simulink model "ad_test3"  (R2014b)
settings: Solver=ode45  StartTime=0.0  StopTime=10  MaxStep=1e-4  RelTol=1e-3
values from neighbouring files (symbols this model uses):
  ampl = 1    [abtast_rate_1.m]    (also in ad_test_12.m; ad_test_2.m; ad_test_3.m; fft_1.m = 10)
  ampl1 = 1e-4    (= 0.0001)    [ad_test_2.m]    (also in ad_test_3.m; DA_wandler_spektr_1.m = 1; DA_wandler_spektr_2.m = 1; fourier_reihe1.m = 5)
  ampl2 = 1e-5    (= 1e-05)    [ad_test_2.m]    (also in ad_test_3.m; DA_wandler_spektr_1.m = 1; DA_wandler_spektr_2.m = 1; fourier_reihe1.m = 12)
  fsig = 100    [abtast_rate_1.m]    (also in ad_test_12.m = ',num2str(fsig),'; ad_test_2.m = ',num2str(fsig),'; ad_test_3.m = ',num2str(fsig),'; leakage_2.m = 100.5)
  N = 4*1024    (= 4096)    [ad_test_12.m]    (also in ad_test_2.m; ad_test_3.m; DA_wandler_spektr_1.m = 1000; DA_wandler_spektr_2.m = 1024)
  Ts = 1/fs    (= 0.00025)    [abtast_rate_1.m]    (also in ad_test_12.m = 0.0009765625; ad_test_2.m = 0.00048828125; ad_test_3.m = 0.00048828125; DA_wandler_spektr_1.m = 0.01)
undefined symbols (not defined in the file or in its folder): get
libraries: dspspect3 x1, dspstat3 x1, dspsnks4 x1, dspsigops x1

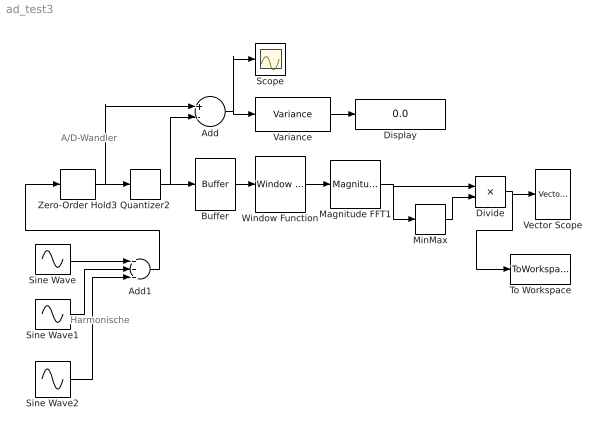
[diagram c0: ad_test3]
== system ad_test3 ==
  note: Harmonische
  note: A/D-Wandler
  Add : Sum  Inputs=+-
  Add1 : Sum  Inputs=+++  SampleTime=0
  Buffer : Buffer  N=N  TreatMby1Signals=One channel
  Display : Display
  Divide : Product  Inputs=*/
  Magnitude FFT1 : dspspect3/Magnitude FFT  mag_or_magsq=Magnitude squared  FFTImplementation=FFTW  fftLenInherit=off  fftsize=N  WrapInput=on
  MinMax : MinMax  Function=max  OutDataTypeStr=double
  Quantizer2 : Quantizer  QuantizationInterval=q  LinearizeAsGain=off  SampleTime=Ts
  Scope : Scope
  Sine Wave : Sin  Amplitude=ampl  Frequency=2*pi*fsig  SampleTime=0
  Sine Wave1 : Sin  Amplitude=ampl1  Frequency=2*pi*[2*fsig]  SampleTime=0
  Sine Wave2 : Sin  Amplitude=ampl2  Frequency=2*pi*[3*fsig]  SampleTime=0
  To Workspace : ToWorkspace  VariableName=Y  SampleTime=-1
  Variance : dspstat3/Variance  run=on  reset_popup=None  InputProcessing=Columns as channels (frame based)  directionMode=Each column  dimension=1  treatSBRowAsCol=on  roiEnable=off  roiType=Rectangles  roiPortion=Entire ROI  roiOutput=Individual statistics for each ROI  roiFlag=off  roundingMode=Floor  overflowMode=off
  Vector Scope : dspsnks4/Vector Scope  ScopeProperties=on  Domain=Frequency  HorizSpan=1  DisplayProperties=off  AxisGrid=on  Memory=off  FrameNumber=on  AxisLegend=off  AxisZoom=off  OpenScopeAtSimStart=on  OpenScopeImmediately=off  FigPos=get(0,'defaultfigureposition')  AxisProperties=off  XUnits=Hertz  XRange=[0...Fs]  InheritXIncr=on  XIncr=1  XLabel=Time  XLimit=User-defined  XMin=2.1333  XMax=2050.1333  XStart=0  YUnits=dB  YLabel=Leistung in dB  LineProperties=off  XAxisParamsVer=6.9
  Window Function : dspsigops/Window Function  winmode=Apply window to input  wintype=Hanning  sampmode=Continuous  samptime=1  N=64  Rs=50  beta=10  winsamp=Symmetric  UserWindow=hamming  OptParams=off  UserParams={'symmetric'}  RowConvenienceOn=on  dataType=double  isSigned=on  wordLen=16  udDataType=sfix(16)  fracBitsMode=Best precision  numFracBits=15  roundingMode=Floor  overflowMode=off  numSidelobes=4  sidelobeLevel=-30
  Zero-Order Hold3 : ZeroOrderHold  SampleTime=Ts
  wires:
  Buffer/1 -> Window Function/1
  Variance/1 -> Display/1
  Magnitude FFT1/1 -> MinMax/1, Divide/1
  Divide/1 -> Vector Scope/1, To Workspace/1
  MinMax/1 -> Divide/2
  Add/1 -> Scope/1, Variance/1
  Zero-Order Hold3/1 -> Quantizer2/1, Add/1
  Quantizer2/1 -> Add/2, Buffer/1
  Add1/1 -> Zero-Order Hold3/1
  Sine Wave/1 -> Add1/1
  Sine Wave1/1 -> Add1/2
  Sine Wave2/1 -> Add1/3
  Window Function/1 -> Magnitude FFT1/1
